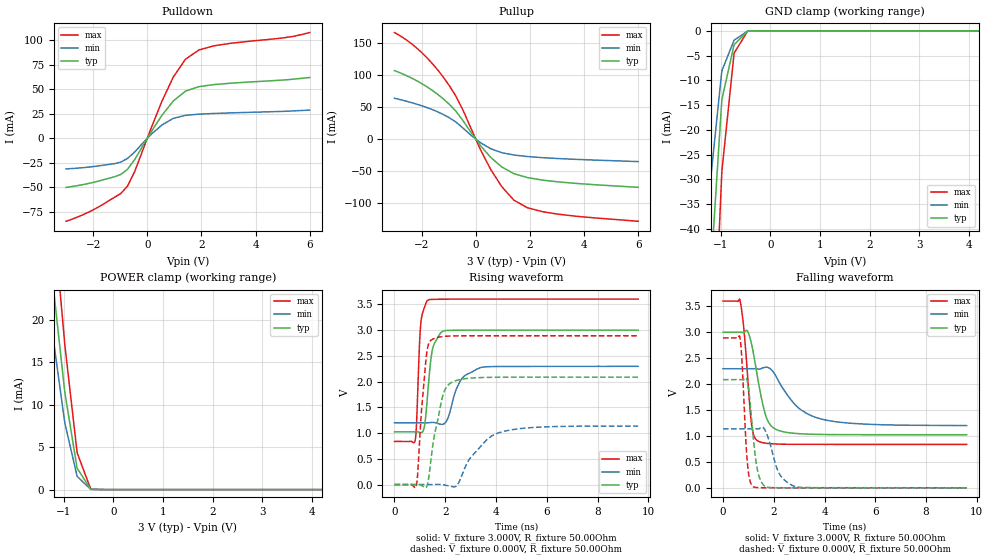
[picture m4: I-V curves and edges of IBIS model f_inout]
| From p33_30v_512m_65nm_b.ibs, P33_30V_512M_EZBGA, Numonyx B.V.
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[Model]   f_inout
Model_type   I/O
Vinl = 0.400V
Vinh = 2.600V
Vmeas = 1.500V
Cref = 30.000pF
|   typ   min   max
C_comp   2.380pF   2.200pF   2.540pF
[Voltage Range]   3.000V   2.300V   3.600V
[Temperature Range]   25.0   85.0   -40.0
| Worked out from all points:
|   slope of the pulldown table from 0 to 0.45 V, typ, clamps not added: 22.9 ohm
|   slope of the pullup table from 0 to 0.45 V, typ, clamps not added: 19 ohm
|   falling waveform, V_fixture 3.000V, R_fixture 50.00Ohm: 20-80 % time 472ps typ, 1.19ns min, 263ps max; typ from 3 V to 1.02 V
|   rising waveform, V_fixture 3.000V, R_fixture 50.00Ohm: 20-80 % time 239ps typ, 497ps min, 137ps max; typ from 1.02 V to 3 V
|   rising waveform, V_fixture 0.000V, R_fixture 50.00Ohm: 20-80 % time 453ps typ, 1.05ns min, 260ps max; typ from 0.002 V to 2.08 V
|   falling waveform, V_fixture 0.000V, R_fixture 50.00Ohm: 20-80 % time 266ps typ, 461ps min, 182ps max; typ from 2.08 V to 0.002 V
[Pulldown]
|   Voltage   I(typ)   I(min)   I(max)
-3V       -50.1mA    -31.2mA    -84.69mA
-1.749V   -43.27mA   -27.94mA   -69.27mA
-984mV    -36.96mA   -24.3mA    -56.43mA
-732mV    -31.69mA   -20.61mA   -48.94mA
-453mV    -21.26mA   -13.64mA   -33.22mA
555mV     23.93mA    13.82mA    38.6mA
960mV     38.04mA    20.32mA    62.39mA
1.41V     48.08mA    23.44mA    80.66mA
1.905V    52.69mA    24.65mA    90.12mA
2.454V    54.82mA    25.37mA    94.37mA
5.055V    59.58mA    27.57mA    102.7mA
6V        62.1mA     28.85mA    108mA
[GND Clamp]
|   Voltage   I(typ)   I(min)   I(max)
-3V       -494.6mA   -417.3mA   -598mA
-1.344V   -80.07mA   -54.28mA   -119.1mA
-1.209V   -50.67mA   -31.14mA   -82.66mA
-1.2V     -48.79mA   -29.7mA    -80.28mA
-984mV    -14.86mA   -8.664mA   -29.88mA
-975mV    -13.8mA    -8.017mA   -28.22mA
-732mV    -2.859mA   -1.927mA   -4.658mA
-723mV    -2.716mA   -1.839mA   -4.39mA
-453mV    -33.1uA    -41.97uA   -18.74uA
6V        0A         0A         0A
[Pullup]
|   Voltage   I(typ)   I(min)   I(max)
-3V       107.1mA    63.94mA    166.5mA
-2.028V   87.66mA    52.68mA    136.6mA
-1.2V     63.04mA    38.61mA    97.04mA
-723mV    43.24mA    26.49mA    66.51mA
-453mV    27.94mA    16.73mA    43.75mA
177mV     -10.08mA   -5.555mA   -16.48mA
546mV     -28.07mA   -14.71mA   -46.7mA
960mV     -43.32mA   -21.09mA   -73.99mA
1.41V     -53.83mA   -24.72mA   -95.27mA
1.905V    -59.91mA   -27.08mA   -107mA
2.454V    -63.84mA   -28.86mA   -113.2mA
6V        -75.24mA   -35.03mA   -128.3mA
[POWER Clamp]
|   Voltage   I(typ)   I(min)   I(max)
-3V       146.8mA    123.2mA    174.1mA
-1.344V   31.97mA    24.47mA    41.98mA
-1.209V   23.84mA    17.71mA    32.31mA
-1.2V     23.3mA     17.27mA    31.68mA
-984mV    11.76mA    8.086mA    17.42mA
-975mV    11.33mA    7.758mA    16.87mA
-732mV    2.57mA     1.599mA    4.416mA
-453mV    30.18uA    19.57uA    45.89uA
6V        0A         0A         0A
[Ramp]
R_load = 50.00Ohm
|   typ   min   max
dV/dt_r   1.250V/453.185ps 680.579mV/1.045ns   1.732V/260.208ps
dV/dt_f   1.183V/471.655ps 656.655mV/1.191ns   1.656V/262.641ps
[Falling Waveform]
V_fixture = 3.000V
V_fixture_min = 2.300V
V_fixture_max = 3.600V
R_fixture = 50.00Ohm
|   Time   V(typ)   V(min)   V(max)
0s        2.996V     2.294V     3.597V
670ps     2.996V     2.294V     3.614V
830ps     2.99V      2.294V     3.025V
1.12ns    2.782V     2.294V     1.25V
1.36ns    2.134V     2.293V     907.8mV
1.76ns    1.298V     2.32V      856.8mV
2.33ns    1.086V     1.938V     841.9mV
3.09ns    1.042V     1.498V     838.5mV
4.09ns    1.028V     1.302V     838mV
9.6ns     1.024V     1.2V       837.9mV
[Rising Waveform]
V_fixture = 3.000V
V_fixture_min = 2.300V
V_fixture_max = 3.600V
R_fixture = 50.00Ohm
|   Time   V(typ)   V(min)   V(max)
0s        1.024V     1.2V       837.9mV
810ps     1.024V     1.2V       846.2mV
1.04ns    1.009V     1.2V       3.141V
1.2ns     1.199V     1.2V       3.466V
1.35ns    2.013V     1.201V     3.585V
1.53ns    2.683V     1.207V     3.593V
1.96ns    2.983V     1.182V     3.596V
2.62ns    2.994V     2.032V     3.597V
3.39ns    2.996V     2.271V     3.597V
9.6ns     2.996V     2.294V     3.597V
[Rising Waveform]
V_fixture = 0.000V
V_fixture_min = 0.000V
V_fixture_max = 0.000V
R_fixture = 50.00Ohm
|   Time   V(typ)   V(min)   V(max)
0s        1.602mV    3.038mV    1.012mV
850ps     2.816mV    3.038mV    -38.59mV
910ps     6.289mV    3.038mV    190.1mV
1.25ns    -52.27mV   2.976mV    2.475V
1.52ns    797.6mV    4.247mV    2.825V
1.97ns    1.823V     -6.045mV   2.875V
2.47ns    2.025V     -8.311mV   2.885V
3ns       2.066V     526.5mV    2.887V
4.09ns    2.083V     1.004V     2.887V
9.6ns     2.085V     1.137V     2.887V
[Falling Waveform]
V_fixture = 0.000V
V_fixture_min = 0.000V
V_fixture_max = 0.000V
R_fixture = 50.00Ohm
|   Time   V(typ)   V(min)   V(max)
0s        2.085V     1.137V     2.887V
670ps     2.085V     1.137V     2.893V
740ps     2.085V     1.137V     2.508V
960ps     2.055V     1.137V     490.1mV
1.19ns    995.9mV    1.137V     23.07mV
1.4ns     257mV      1.135V     5.818mV
1.72ns    17.6mV     1.045V     2.588mV
2.21ns    3.901mV    280.7mV    1.398mV
2.87ns    2.28mV     21.74mV    1.071mV
9.6ns     1.602mV    3.038mV    1.012mV
